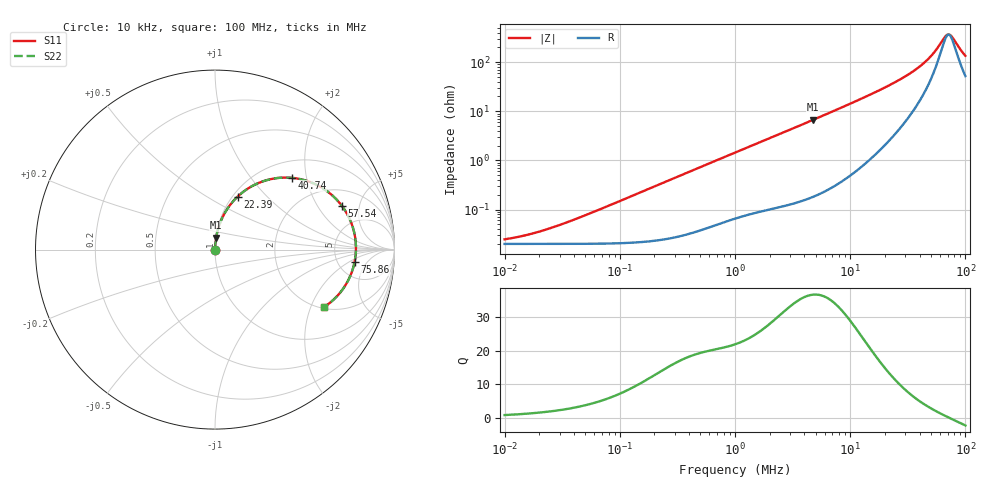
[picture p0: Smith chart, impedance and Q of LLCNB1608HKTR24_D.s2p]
! LLCNB1608HKTR24_D  S-PARAMETER MODEL  ( Standard Model )
! Model Generated by TAIYO YUDEN Corporation (http://www.ty-top.com)
! Version 1.0
! TAIYO YUDEN Control No. 200410
! Copyright(c) 2020 TAIYO YUDEN CO.,LTD. All Rights Reserved.
! Product Description (link to TY-COMPAS)
! https://ds.yuden.co.jp/TYCOMPAS/or/detail?pn=LLCNB1608HKTR24MD&u=M
! Products Name : Inductors
! Characteristics :
!  Inductance : 0.24 [uH] , SRF(min) : - [Hz] , DC Resistance(max) : 24 [mOhm]
!  Rated Current : Saturation  4.3 [A] (dL = 30 [%]), Temp Rise  3.7 [A] (dT = 40 [degC])
!  Case Size : 1.6 x 0.8 / 0.063 x 0.031 [mm/inch] , Thickness : 0.8 / 0.031 [mm/inch]
!  (Conditions: Temperature = 25 [degC] , DC Bias Current = 0 [A])
! External Node Assignments :
!  1  o---GGG---o  2
! GND o---------o GND
! Frequency Range : 10kHz  -  100MHz  [ 402 STEP ]
# MHz S RI R 50
! Freq[MHz].  S11 Real  S11 Imag  S21 Real  S21 Imag  S12 Real  S12 Imag  S22 Real  S22 Imag
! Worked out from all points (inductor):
!   401 points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, 10 kHz to 100 MHz, reference 50 ohm
!   read as one part in series: L = 235 nH near 41.69 kHz
!   highest Q = 36.8 at 4.786 MHz (marker M1), where L = 223 nH
!   self-resonance near 71.55 MHz
!   S11 on the Smith chart (normalised r, x): 10 kHz: 1.00, +0.00; 22.39 MHz: 1.05, +0.69; 40.74 MHz: 1.35, +1.64; 57.54 MHz: 3.06, +3.37; 75.86 MHz: 7.16, -2.60; 100 MHz: 2.04, -2.48
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0.01  0.0002 0.000147  0.9998 -0.000147  0.9998 -0.000147  0.0002 0.000147
0.013804  0.0002 0.000203  0.9998 -0.000203  0.9998 -0.000203  0.0002 0.000203
0.019953  0.0002 0.000294  0.9998 -0.000294  0.9998 -0.000294  0.0002 0.000294
0.046774  0.000201 0.000689  0.9998 -0.000689  0.9998 -0.000689  0.000201 0.000689
0.218776  0.000249 0.00322  0.9998 -0.00322  0.9998 -0.00322  0.000249 0.00322
1  0.000859 0.0143  0.9991 -0.0143  0.9991 -0.0143  0.000859 0.0143
4.677351  0.00605 0.0651  0.994 -0.0651  0.994 -0.0651  0.00605 0.0651
4.786301  0.00629 0.0666  0.9937 -0.0666  0.9937 -0.0666  0.00629 0.0666
12.30269  0.0369 0.1694  0.9631 -0.1694  0.9631 -0.1694  0.0369 0.1694
16.98244  0.0711 0.2307  0.9289 -0.2307  0.9289 -0.2307  0.0711 0.2307
21.87762  0.1204 0.2898  0.8796 -0.2898  0.8796 -0.2898  0.1204 0.2898
22.38721  0.1263 0.2956  0.8737 -0.2956  0.8737 -0.2956  0.1263 0.2956
30.90295  0.2478 0.3733  0.7522 -0.3733  0.7522 -0.3733  0.2478 0.3733
40.73803  0.4272 0.3999  0.5728 -0.3999  0.5728 -0.3999  0.4272 0.3999
48.97788  0.5814 0.353  0.4186 -0.353  0.4186 -0.353  0.5814 0.353
57.54399  0.7084 0.2419  0.2916 -0.2419  0.2916 -0.2419  0.7084 0.2419
66.06934  0.7755 0.0959  0.2245 -0.0959  0.2245 -0.0959  0.7755 0.0959
69.1831  0.7841 0.0408  0.2159 -0.0408  0.2159 -0.0408  0.7841 0.0408
72.4436  0.7848 -0.0153  0.2152 0.0153  0.2152 0.0153  0.7848 -0.0153
75.85776  0.7775 -0.0708  0.2225 0.0708  0.2225 0.0708  0.7775 -0.0708
89.12509  0.697 -0.2403  0.303 0.2403  0.303 0.2403  0.697 -0.2403
100  0.6046 -0.3222  0.3954 0.3222  0.3954 0.3222  0.6046 -0.3222
